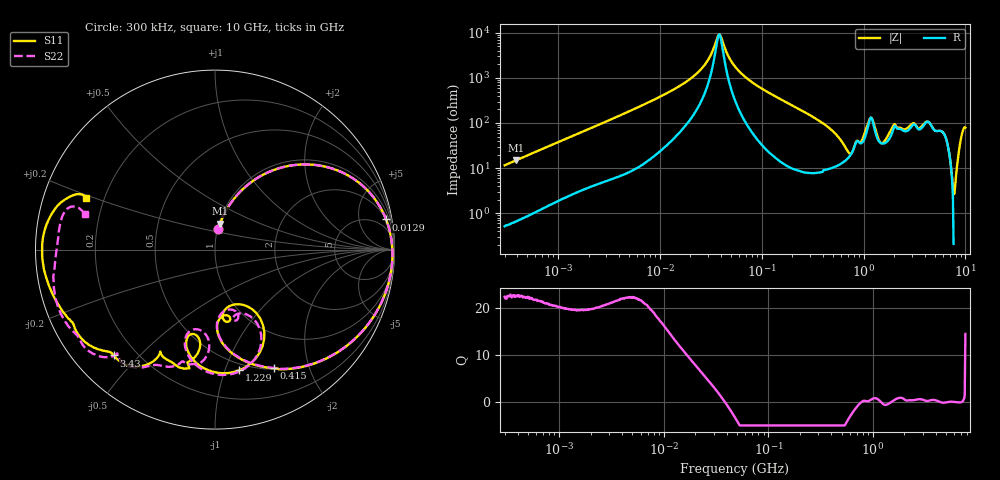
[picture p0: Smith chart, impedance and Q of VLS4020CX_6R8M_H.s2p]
! S-Parameter Data Generated by TDK Corporation
! Copyright(C) 2024 TDK Corporation.
! All Rights Reserved.
! TDK P/N: VLS4020CX-6R8M-H (SMD / SMT Inductor (Coil))
! Property: L=6.8uH at 1MHz
! Size(LxWxT): 4x4x2mm
! Model Type: s2p (Touchstone File Format Version 1.0)
! Frequency: DC=Yes Start=0.3MHz Stop=10000MHz 802points Log-sweep
! Model Generated on May 28, 2024
! Terms and conditions regarding TDK Simulation Models:
! 1)This simulation model is being provided solely for informational
!  purposes. Please refer to the specifications of the products in
!  terms of detailed characteristics of such products.
! 2)In no event shall TDK Corporation of any of its subsidiaries be
!  liable for any loss or damage arising, directly or indirectly,
!  from any information contained in this simulation model, including,
!  but not limited to loss or damages arising from any inaccuracies,
!  omissions or errors in connection with such information.
! 3)Any and all copyrights on this simulation model are owned by
!  TDK Corporation.  Duplication or redistribution of this simulation
!  model without prior written permission from TDK Corporation
!  is prohibited.
! 4)This simulation model is subject to any modification or change
!  without any prior notice.
! 5)Neither TDK Corporation nor any of its subsidiaries shall make any
!  warranty, express or implied, including but not limited to the
!  correctness, implied warranties of merchantability and fitness for
!  a particular purpose with respect to this simulation models.
! 6)The use of this simulation model shall be deemed to have consented
!  to the terms and conditions hereof.
! Port Assignments:
!  1 ---@@@--- 2
! Applicable Conditions:
!  Temperature = 25 degC
!  DC Bias Current = 0 A
!  Small Signal Operation
# Hz S MA R 50
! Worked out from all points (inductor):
!   801 points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, 300 kHz to 10 GHz, reference 50 ohm
!   read as one part in series: L = 6.1 uH near 318.3 kHz
!   highest Q = 22.7 at 391.7 kHz (marker M1), where L = 6.1 uH
!   self-resonance near 38.17 MHz
!   S11 on the Smith chart (normalised r, x): 300 kHz: 1.01, +0.23; 12.9 MHz: 2, +11; 415 MHz: 0.51, -1.49; 1.229 GHz: 0.44, -1.12; 3.43 GHz: 0.12, -0.42; 10 GHz: 0.13, +0.19
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300000  0.1136 80.8  0.9884 -6.6  0.9884 -6.6  0.1136 80.8
391685  0.1469 78.9  0.9827 -8.5  0.9825 -8.5  0.1469 78.9
1713600  0.5216 55.6  0.8269 -31.5  0.827 -31.5  0.5215 55.6
9671944  0.9503 14.4  0.2597 -72.2  0.2597 -72.2  0.9503 14.4
1.289893e7  0.9677 10.0  0.1885 -75.6  0.1885 -75.6  0.9678 10.0
2.599165e7  0.9862 1.7  0.0598 -76.7  0.05982 -76.7  0.9862 1.7
3.817206e7  0.9892 -2.4  0.01078 -6.3  0.01079 -6.2  0.9892 -2.3
5.477226e7  0.9886 -6.6  0.05517 73.2  0.05519 73.2  0.9887 -6.5
1.540638e8  0.9506 -25.6  0.2739 62.2  0.2739 62.1  0.9505 -25.5
3.126428e8  0.8315 -50.7  0.5136 36.7  0.5137 36.7  0.8319 -50.3
4.149731e8  0.7387 -63.5  0.6127 22.3  0.6127 22.3  0.7391 -63.2
6.904357e8  0.4703 -87.9  0.7525 -14.4  0.7526 -14.4  0.4669 -87.9
1.001841e9  0.3261 -69.2  0.644 -51.5  0.6441 -51.6  0.3851 -67.3
1.228555e9  0.686 -78.6  0.3438 -43.6  0.3439 -43.6  0.699 -81.8
1.43752e9  0.6066 -103.2  0.5248 -46.5  0.5252 -46.5  0.5977 -105.1
1.767019e9  0.4905 -101.8  0.5226 -82.0  0.5233 -82.0  0.4594 -99.1
2.112126e9  0.6806 -108.7  0.3281 -88.7  0.3289 -88.8  0.6501 -105.5
3.429941e9  0.8153 -133.7  0.1828 -118.2  0.1823 -118.3  0.795 -133.2
4.34106e9  0.8905 -145.2  0.08731 -125.8  0.08697 -125.7  0.9026 -141.2
5.849356e9  0.9098 -156.6  0.07296 -132.9  0.07292 -132.9  0.9199 -151.9
7.428478e9  0.9627 -176.6  0.05485 -128.6  0.05478 -128.4  0.899 -173.7
1e10  0.7722 158.2  0.0425 -124.7  0.04258 -124.8  0.7508 164.8
